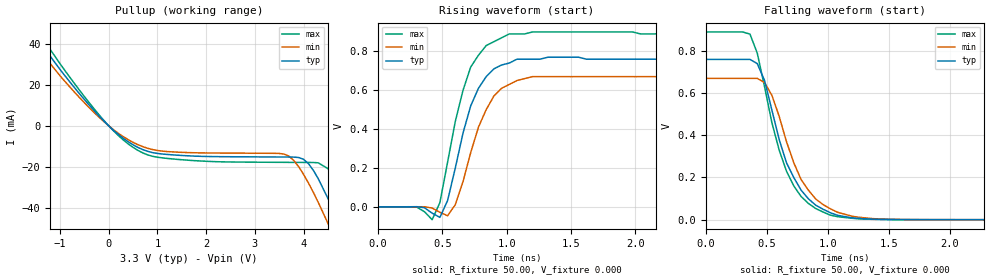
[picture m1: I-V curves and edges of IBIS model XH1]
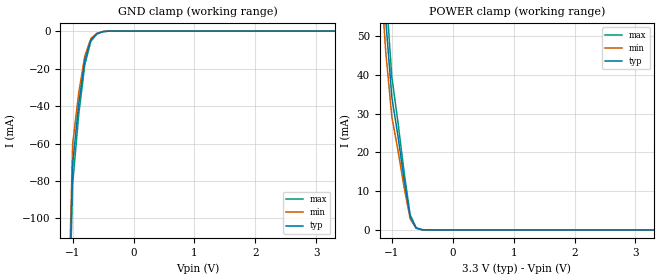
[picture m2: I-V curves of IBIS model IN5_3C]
[IBIS Ver]   2.1
[File name]   557-03.ibs
[File Rev]   1.1
[Date]   7/29/05
[Source]   ICS MicroClock Applications Engineering
[Disclaimer] This information is for modeling purposes only, and is
(C) Copyright Integrated Circuit Systems, Inc. 1997-2005
   All rights reserved
ICS hereby grants the user of this IBIS model a non-exclusive,
nontransferable license to use this IBIS model under the following terms.
Before using this IBIS model, the user should read this license.
If the user does not accept these terms,  the IBIS model should be
returned to ICS within 30 days.
   The user is granted this license only to use the IBIS model and
is not granted rights to sell, load, rent, lease or license the IBIS
model in whole or in part, or in modified form to anyone other than
user. User may modify the IBIS model to suit its specific
applications but rights to derivative works and such modifications
shall belong to ICS.
   This IBIS model is provided on an "AS IS" basis and ICS makes
absolutely no warranty with respect to the information contained
herein. ICS DISCLAIMS AND CUSTOMER WAIVES ALL WARRANTIES, EXPRESS
OR IMPLIED, INCLUDING WARRANTIES OF MERCHANTABILITY OR FITNESS FOR
A PARTICULAR PURPOSE. The entire risk as to quality and performance
is with the Customer. ACCORDINGLY, IN NO EVENT SHALL THE COMPANY BE
LIABLE FOR ANY DAMAGES, WHETHER IN CONTRACT OR TORT,INCLUDING ANY
LOST PROFITS OR OTHER INCIDENTAL, CONSEQUENTIAL, EXEMPLARY, OR
PUNITIVE DAMAGES ARISING OUT OF THE USE OR APPLICATION OF THE IBIS
model provided in this package. Further, ICS reserves the right to
make changes without notice to any product herein to improve
reliability, function, or design. ICS does not convey any license
under patent rights or any other intellectual property rights,
including those of third parties.
   ICS is not obligated to provide maintenance or support
for the licensed IBIS model.
[Component]   ICS557-03
[Manufacturer] Integrated Circuit Systems Inc.
[Package]
|   typ   min   max
R_pkg   57.05m   55.5m   58.6m
L_pkg   1.769nH   1.57nH   1.968nH
C_pkg   0.269pF   0.252pF   0.286pF
[pin]   signal_name   model_name   R_pin   L_pin   C_pin
   1   S0   IN5_3C   86m   2n   86f
   2   S1   IN5_3C   86m   2n   86f
   3   SS0   IN5_3C   76m   1.8n   77f
   4   X1/ICLK   IN5_3C   62m   1.4n   62f
   6   OE   IN5_3C   65m   1.5n   65f
   8   SS1   IN5_3C   89m   2n   89f
  10   /CLK1   XH1   86m   2n   86f
  11   CLK1   XH1   71m   1.6n   71f
  14   /CLK0   XH1   71m   1.6n   71f
  15   CLK0   XH1   86m   2n   86f
[Diff Pin]  inv_pin  vdiff   tdelay_typ  tdelay_min  tdelay_max
11   10   0.000V   0.000s   0.000s   0.000s
15   14   0.000V   0.000s   0.000s   0.000s
| Models and submodels in the file (2): XH1 (Open_source), IN5_3C (Input)
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|   Model XH1
[Model]   XH1
Model_type   Open_source
Polarity   Inverting
Vmeas =  0.35000V
Rref = 50.00000
Vref =  0.000V
C_comp   3.40pF   2.85pF   3.95pF
[Temperature Range]   25.00   70.00   0.000
[Voltage Range]   3.30V   3.00V   3.70V
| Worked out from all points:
|   slope of the pullup table from 0 to 0.495 V, typ, clamps not added: 53.7 ohm
|   rising waveform, R_fixture 50.00, V_fixture 0.000: 20-80 % time 196ps typ, 209ps min, 191ps max; typ from 0 V to 0.76 V
|   falling waveform, R_fixture 50.00, V_fixture 0.000: 20-80 % time 266ps typ, 276ps min, 255ps max; typ from 0.76 V to 0 V
[Pullup]
| voltage   I(typ)   I(min)   I(max)
-3.3V     120mA      110mA      120mA
-1.9V     57.97mA    52.49mA    62.98mA
-1.5V     43.73mA    39.31mA    47.78mA
-100mV    2.37mA     2.07mA     2.66mA
700mV     -11.65mA   -10.21mA   -13.27mA
3.6V      -15.27mA   -13.83mA   -17.88mA
4V        -16.4mA    -23.77mA   -17.93mA
4.3V      -25.83mA   -37.4mA    -18.11mA
4.5V      -35.53mA   -47.74mA   -20.97mA
4.7V      -46.5mA    -58.63mA   -28.65mA
5.1V      -70.24mA   -81.19mA   -50.61mA
6.6V      -160mA     -170mA     -150mA
[Ramp]
| variable   typ   min   max
dV/dt_r   0.46/0.20n   0.40/0.21n   0.53/0.19n
dV/dt_f   0.45/0.26n   0.40/0.27n   0.53/0.25n
R_load = 50.00
[Rising Waveform]
R_fixture = 50.00
V_fixture = 0.000
V_fixture_min = 0.000
V_fixture_max = 0.000
| time   V(typ)   V(min)   V(max)
0s        -370nV     -380nV     -340nV
300ps     550uV      230uV      -1.44mV
420ps     -32.86mV   -6.35mV    -66.34mV
480ps     -54.44mV   -28.27mV   21.55mV
540ps     32.24mV    -46.01mV   230mV
600ps     200mV      10.91mV    440mV
720ps     520mV      280mV      720mV
840ps     670mV      500mV      830mV
1.02ns    740mV      630mV      890mV
3ns       760mV      670mV      890mV
[Falling Waveform]
R_fixture = 50.00
V_fixture = 0.000
V_fixture_min = 0.000
V_fixture_max = 0.000
| time   V(typ)   V(min)   V(max)
0s        760mV      670mV      890mV
360ps     760mV      670mV      880mV
420ps     740mV      670mV      790mV
480ps     660mV      650mV      630mV
540ps     520mV      590mV      460mV
660ps     270mV      370mV      230mV
780ps     140mV      190mV      110mV
900ps     68.75mV    97.98mV    52.94mV
1.38ns    2.27mV     4.59mV     1.49mV
3ns       -13.74uV   -37.6uV    -15.05uV
[Model]   IN5_3C
Model_type   Input
|   typ   min   max
C_comp   5pF   4pF   6pF
Vinl =1.15V   | Input logic  "low" DC voltage
Vinh=2.15V   | Input logic  "high" DC voltage
|   typ   min   max
[Voltage range]  3.3V   2.97V   3.63V
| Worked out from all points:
|   GND clamp passes 1 mA (typ) near -0.57 V on its own axis
|   POWER clamp passes 1 mA (typ) near -0.62 V on its own axis
[GND_clamp]
|Voltage I (typ)   I (min)   I (max)
-3.3V     -3A        -3A        -3A
-1V       -70.99mA   -60.34mA   -81.64mA
-900mV    -38.73mA   -32.92mA   -44.54mA
-800mV    -15.56mA   -13.23mA   -17.89mA
-700mV    -4.62mA    -3.92mA    -5.31mA
-600mV    -1.36mA    -1.16mA    -1.57mA
-500mV    -260uA     -220uA     -300uA
-400mV    -24.9uA    -21uA      -29uA
3.3V      858nA      729nA      986nA
[POWER_clamp]
|Voltage I (typ)   I (min)   I (max)
-3.3V     3A         3A         3A
-1.2V     81.31mA    69.12mA    93.51mA
-1.1V     54.18mA    46.05mA    62.31mA
-1V       34.31mA    29.17mA    39.46mA
-900mV    24.27mA    20.63mA    27.91mA
-800mV    13.12mA    11.15mA    15.08mA
-700mV    3.44mA     2.924mA    3.956mA
-600mV    472uA      401uA      543uA
-500mV    50.5uA     42.9uA     58.1uA
-400mV    6.01uA     5.1uA      6.91uA
3.3V      -5.78uA    -4.9uA     -6.6uA
